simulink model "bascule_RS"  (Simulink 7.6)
settings: Solver=ode15s  StartTime=0.0  StopTime=1  RelTol=1e-3
libraries: fl_lib x6, nesl_utility x4, elec_lib x2

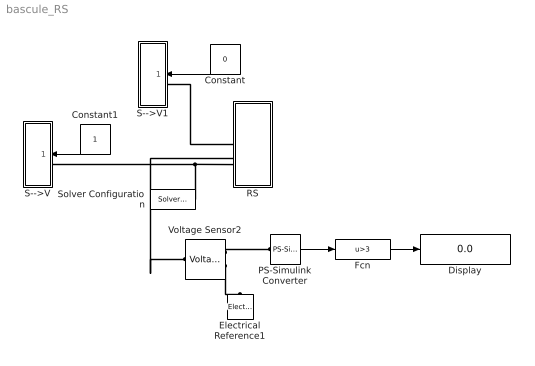
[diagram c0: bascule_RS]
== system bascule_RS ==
  Constant : Constant  Value=0
  Constant1 : Constant
  Display : Display
  Electrical Reference1 : fl_lib/Electrical/Electrical Elements/Electrical Reference  DialogController=NetworkEngine.DynNeDlgSource  SystemSampleTime=-1  i_Log=off  LocalVarNames=|i  LocalVarDescs=|i  LocalVarLogging=[]
  Fcn : Fcn  Expr=u>3
  PS-Simulink Converter : nesl_utility/PS-Simulink Converter  DialogController=NetworkEngine.DynNeUtilDlgSource  SystemSampleTime=-1  PhysicalDomain=network_engine_domain  LeftPortType=input  RightPortType=output  SubClassName=ps_output  Unit=1  AffineConversion=off
  RS : Subsystem
  S-->V : Subsystem
  S-->V1 : Subsystem
  Solver Configuration : nesl_utility/Solver Configuration  DialogController=NetworkEngine.DynNeUtilDlgSource  SystemSampleTime=-1  PhysicalDomain=network_engine_domain  LeftPortType=input  RightPortType=generic  SubClassName=solver  Accelerate=off  Profile=off  ResidualTolerance=1e-9  MaxNonlinIter=12  MaxModeIter=2  DoFixedCost=off  UseLocalSampling=off  DoDC=off  LinearAlgebra=Sparse  LocalSolverSampleTime=.001  LocalSolverChoice=NE_BACKWARD_EULER_ADVANCER  UseLocalSolver=off
  Voltage Sensor2 : fl_lib/Electrical/Electrical Sensors/Voltage Sensor  DialogController=NetworkEngine.DynNeDlgSource  SystemSampleTime=-1  i1_Log=off  v1_Log=off  LocalVarNames=|i1|v1  LocalVarDescs=|i1|v1  LocalVarLogging=[]
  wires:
  PS-Simulink Converter/1 -> Fcn/1
  Constant/1 -> S-->V1/1(S1)
  Constant1/1 -> S-->V/1(S1)
  Fcn/1 -> Display/1
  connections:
  Voltage Sensor2/RConn1 -- PS-Simulink Converter/LConn1
  RS/LConn2 -- Voltage Sensor2/LConn1
  Voltage Sensor2/RConn2 -- Electrical Reference1/LConn1
  S-->V1/LConn1 -- RS/LConn1
  S-->V/LConn1 -- RS/LConn3 -- Solver Configuration/RConn1

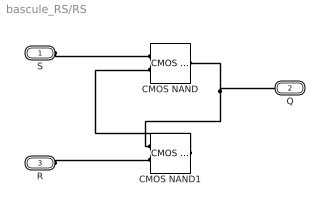
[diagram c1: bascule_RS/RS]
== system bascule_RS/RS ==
  CMOS NAND : elec_lib/Integrated Circuits/Logic/CMOS NAND  DialogController=NetworkEngine.DynNeDlgSource  SystemSampleTime=-1  V_IL=2 V  V_IH=3 V  C_IN=5 pF  output_type=1  V_OL=0 V  V_OH=5 V  V_CC=5 V  V_meas=5 V  R_OUT=450 Ohm  R_OH=[ 25 250 ] Ohm  I_OH=63 mA  R_OL=[ 30 800 ] Ohm  I_OL=-45 mA  Delay=1.2e-07 s  Ron=5 Ohm  Vf=0.6 V  output_state=1  LocalVarLogging=[]
  CMOS NAND1 : elec_lib/Integrated Circuits/Logic/CMOS NAND  DialogController=NetworkEngine.DynNeDlgSource  SystemSampleTime=-1  V_IL=2 V  V_IH=3 V  C_IN=5 pF  output_type=1  V_OL=0 V  V_OH=5 V  V_CC=5 V  V_meas=5 V  R_OUT=450 Ohm  R_OH=[ 25 250 ] Ohm  I_OH=63 mA  R_OL=[ 30 800 ] Ohm  I_OL=-45 mA  Delay=1.2e-07 s  Ron=5 Ohm  Vf=0.6 V  output_state=1  LocalVarLogging=[]
  S : PMIOPort  Port=1  Side=Left
  Q : PMIOPort  Port=2  Side=Left
  R : PMIOPort  Port=3  Side=Left
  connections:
  S/RConn1 -- CMOS NAND/LConn1
  CMOS NAND1/RConn1 -- CMOS NAND/LConn2
  CMOS NAND1/LConn1 -- CMOS NAND/RConn1 -- Q/RConn1
  R/RConn1 -- CMOS NAND1/LConn2

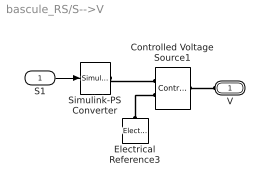
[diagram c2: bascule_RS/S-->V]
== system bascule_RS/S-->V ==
  S1 : Inport
  Controlled Voltage Source1 : fl_lib/Electrical/Electrical Sources/Controlled Voltage Source  DialogController=NetworkEngine.DynNeDlgSource  SystemSampleTime=-1  i_Log=off  v_Log=off  LocalVarNames=|current|voltage|power  LocalVarDescs=|Current (A)|Voltage (V)|Power (W)  LocalVarLogging=[0 0 0]
  Electrical Reference3 : fl_lib/Electrical/Electrical Elements/Electrical Reference  DialogController=NetworkEngine.DynNeDlgSource  SystemSampleTime=-1  i_Log=off  LocalVarNames=|i  LocalVarDescs=|i  LocalVarLogging=[]
  Simulink-PS Converter : nesl_utility/Simulink-PS Converter  DialogController=NetworkEngine.DynNeUtilDlgSource  SystemSampleTime=-1  PhysicalDomain=network_engine_domain  LeftPortType=input  RightPortType=output  SubClassName=ps_input  Unit=1  AffineConversion=off  InputFilterTimeConstant=.001  UdotUserProvided=0
  V : PMIOPort  Port=1  Side=Left
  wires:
  S1/1 -> Simulink-PS Converter/1
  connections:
  Electrical Reference3/LConn1 -- Controlled Voltage Source1/RConn2
  V/RConn1 -- Controlled Voltage Source1/LConn1
  Simulink-PS Converter/RConn1 -- Controlled Voltage Source1/RConn1

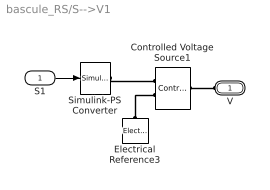
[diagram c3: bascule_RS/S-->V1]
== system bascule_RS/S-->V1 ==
  S1 : Inport
  Controlled Voltage Source1 : fl_lib/Electrical/Electrical Sources/Controlled Voltage Source  DialogController=NetworkEngine.DynNeDlgSource  SystemSampleTime=-1  i_Log=off  v_Log=off  LocalVarNames=|current|voltage|power  LocalVarDescs=|Current (A)|Voltage (V)|Power (W)  LocalVarLogging=[0 0 0]
  Electrical Reference3 : fl_lib/Electrical/Electrical Elements/Electrical Reference  DialogController=NetworkEngine.DynNeDlgSource  SystemSampleTime=-1  i_Log=off  LocalVarNames=|i  LocalVarDescs=|i  LocalVarLogging=[]
  Simulink-PS Converter : nesl_utility/Simulink-PS Converter  DialogController=NetworkEngine.DynNeUtilDlgSource  SystemSampleTime=-1  PhysicalDomain=network_engine_domain  LeftPortType=input  RightPortType=output  SubClassName=ps_input  Unit=1  AffineConversion=off  InputFilterTimeConstant=.001  UdotUserProvided=0
  V : PMIOPort  Port=1  Side=Left
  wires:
  S1/1 -> Simulink-PS Converter/1
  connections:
  Simulink-PS Converter/RConn1 -- Controlled Voltage Source1/RConn1
  V/RConn1 -- Controlled Voltage Source1/LConn1
  Electrical Reference3/LConn1 -- Controlled Voltage Source1/RConn2
